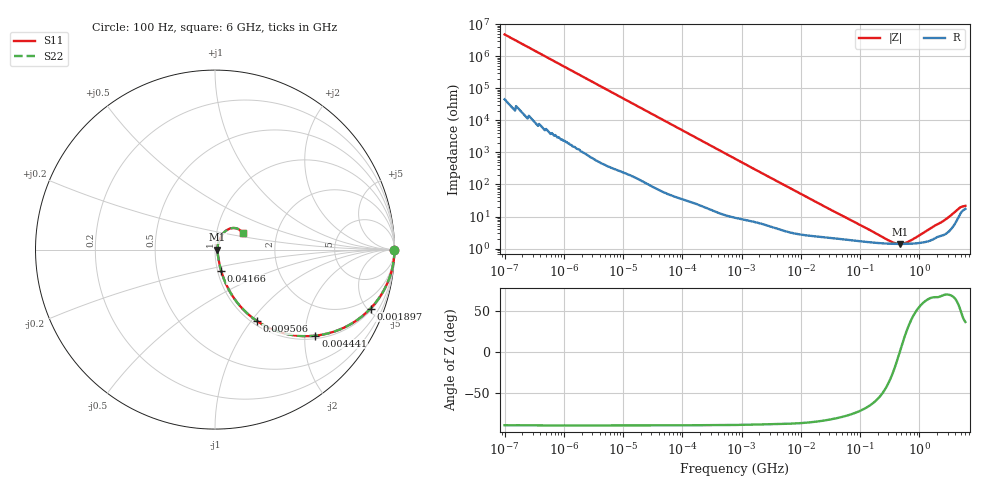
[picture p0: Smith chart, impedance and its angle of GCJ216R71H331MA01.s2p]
!Murata Part Number: GCJ216R71H331MA01
!These Parameters are Measured in Series Mode Connection
!Data Generated on Mar 13, 2026
!  o--ll--o
!Port1  Port2
!  o------o
!Operation Temp=25[degC], DC Bias Voltage=0[V]
!Freq. Start=100[Hz] Stop=6[GHz] 401[Steps]
# Hz S RI R 50
!Freq.(Hz) S11(Real) S11(Imag) S21(Real) S21(Imag) S12(Real) S12(Imag) S22(Real) S22(Imag)
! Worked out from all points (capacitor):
!   401 points, 100 Hz to 6 GHz, reference 50 ohm
!   read as one part in series: C = 334 pF near 109 Hz
!   lowest |Z| = 1.4 ohm at 467.5 MHz (marker M1)
!   series resonance near 469.8 MHz, so ESL is about 340 pH
!   S11 on the Smith chart (normalised r, x): 100 Hz: open; 1.897 MHz: 1.13, -5.23; 4.441 MHz: 1.08, -2.26; 9.506 MHz: 1.06, -1.06; 41.66 MHz: 1.04, -0.25; 6 GHz: 1.35, +0.25
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100  1 -2.1e-05  2e-07 2.1e-05  2e-07 2.1e-05  1 -2.1e-05
479  1 -0.0001  5e-07 0.0001  5e-07 0.0001  1 -0.0001
2008  1 -0.000417  2e-06 0.000417  2e-06 0.000417  1 -0.000417
40335  0.9999 -0.00831  0.000115 0.00831  0.000115 0.00831  0.9999 -0.00831
241822  0.9971 -0.0493  0.0029 0.0493  0.0029 0.0493  0.9971 -0.0493
774597  0.9737 -0.153  0.0263 0.153  0.0263 0.153  0.9737 -0.153
1896632  0.8664 -0.3283  0.1336 0.3283  0.1336 0.3283  0.8664 -0.3283
2837864  0.7493 -0.4191  0.2507 0.4191  0.2507 0.4191  0.7493 -0.4191
4440638  0.5592 -0.4795  0.4408 0.4795  0.4408 0.4795  0.5592 -0.4795
6353432  0.3909 -0.468  0.6091 0.468  0.6091 0.468  0.3909 -0.468
9506416  0.2327 -0.3973  0.7673 0.3973  0.7673 0.3973  0.2327 -0.3973
1.555665e7  0.1142 -0.2827  0.8858 0.2827  0.8858 0.2827  0.1142 -0.2827
4.165952e7  0.0344 -0.1179  0.9656 0.1179  0.9656 0.1179  0.0344 -0.1179
9.753859e7  0.0194 -0.0515  0.9806 0.0515  0.9806 0.0515  0.0194 -0.0515
3.124326e8  0.0141 -0.00999  0.9859 0.00999  0.9859 0.00999  0.0141 -0.00999
3.908258e8  0.0139 -0.00444  0.9861 0.00444  0.9861 0.00444  0.0139 -0.00444
4.674818e8  0.0138 -0.000118  0.9862 0.000118  0.9862 0.000118  0.0138 -0.000118
5.847788e8  0.0139 0.00535  0.9861 -0.00535  0.9861 -0.00535  0.0139 0.00535
7.31507e8  0.0142 0.0111  0.9858 -0.0111  0.9858 -0.0111  0.0142 0.0111
3.065283e9  0.0383 0.081  0.9617 -0.081  0.9617 -0.081  0.0383 0.081
4.586474e9  0.1028 0.1206  0.8972 -0.1206  0.8972 -0.1206  0.1028 0.1206
6e9  0.158 0.0913  0.842 -0.0913  0.842 -0.0913  0.158 0.0913
